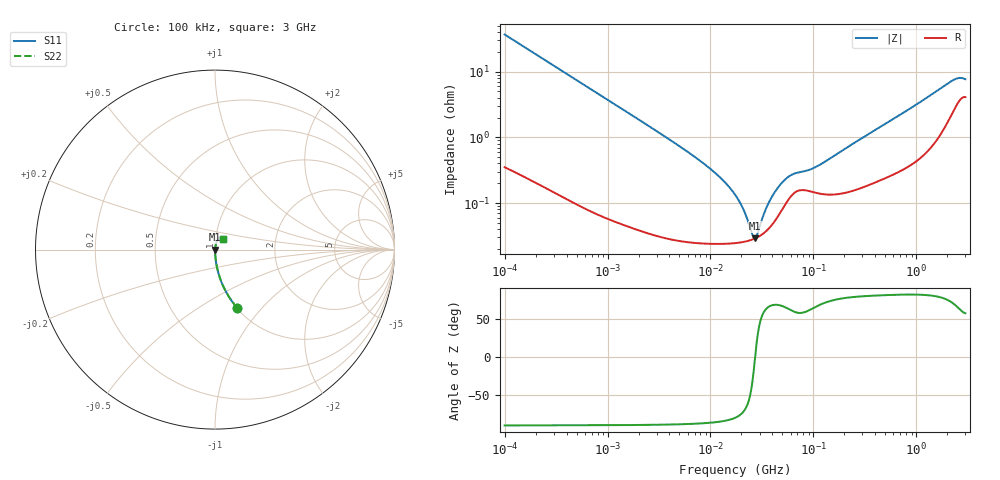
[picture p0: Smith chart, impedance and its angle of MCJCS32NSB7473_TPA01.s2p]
! MCJCS32NSB7473_TPA01  S-PARAMETER MODEL  ( Standard Model )
! Model Generated by TAIYO YUDEN Corporation (http://www.ty-top.com)
! Version 1.0
! TAIYO YUDEN Control No. 220601
! Copyright(c) 2015 TAIYO YUDEN CO.,LTD. All Rights Reserved.
! Product Description (link to TY-COMPAS)
! https://ds.yuden.co.jp/TYCOMPAS/or/detail?pn=MCJCS32NSB7473KTPA01&u=M
! Products Name : Multilayer Ceramic Capacitors
! Characteristics :
!  Capacitance : 0.047 [uF] , Rated Voltage : 630 [V] , TCC : X7R
!  Case Size : 3.2 x 2.5 / 0.126 x 0.098 [mm/inch] , Thickness : 1.9 / 0.075 [mm/inch]
!  (Conditions: Temperature = 25 [degC] , DC Bias Voltage = 0 [V])
! External Node Assignments :
!  1  o---| |---o  2
! GND o---------o GND
! Frequency Range : 100kHz  -  3GHz  [ 401 STEP ]
# MHZ S RI R 50
! Freq[MHz].  S11 Real  S11 Imag  S21 Real  S21 Imag  S12 Real  S12 Imag  S22 Real  S22 Imag
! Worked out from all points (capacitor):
!   401 points, 100 kHz to 3 GHz, reference 50 ohm
!   read as one part in series: C = 43 nF near 105.3 kHz
!   lowest |Z| = 28.8 mohm at 26.84 MHz (marker M1)
!   series resonance near 27.15 MHz, so ESL is about 800 pH
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0.1  0.1224 -0.323  0.8776 0.323  0.8776 0.323  0.1224 -0.323
0.234079  0.0262 -0.1543  0.9738 0.1543  0.9738 0.1543  0.0262 -0.1543
0.562235  0.00525 -0.0661  0.9947 0.0661  0.9947 0.0661  0.00525 -0.0661
3.161081  0.000447 -0.0118  0.9996 0.0118  0.9996 0.0118  0.000447 -0.0118
6.3393  0.000282 -0.00566  0.9997 0.00566  0.9997 0.00566  0.000282 -0.00566
10.08119  0.000249 -0.00326  0.9998 0.00326  0.9998 0.00326  0.000249 -0.00326
14.09348  0.000243 -0.00199  0.9998 0.00199  0.9998 0.00199  0.000243 -0.00199
17.7727  0.000247 -0.00124  0.9998 0.00124  0.9998 0.00124  0.000247 -0.00124
20.74485  0.000255 -0.00078  0.9997 0.00078  0.9997 0.00078  0.000255 -0.00078
25.49486  0.000277 -0.000183  0.9997 0.000183  0.9997 0.000183  0.000277 -0.000183
26.84345  0.000286 -3.32e-05  0.9997 3.32e-05  0.9997 3.32e-05  0.000286 -3.32e-05
28.26337  0.000297 0.000117  0.9997 -0.000117  0.9997 -0.000117  0.000297 0.000117
32.98988  0.000347 0.00058  0.9997 -0.00058  0.9997 -0.00058  0.000347 0.00058
37.52708  0.000421 0.000984  0.9996 -0.000984  0.9996 -0.000984  0.000421 0.000984
42.68829  0.000546 0.0014  0.9995 -0.0014  0.9995 -0.0014  0.000546 0.0014
48.55934  0.000749 0.00182  0.9993 -0.00182  0.9993 -0.00182  0.000749 0.00182
62.83488  0.00135 0.00238  0.9987 -0.00238  0.9987 -0.00238  0.00135 0.00238
97.38194  0.00148 0.00298  0.9985 -0.00298  0.9985 -0.00298  0.00148 0.00298
547.5153  0.00283 0.0172  0.9972 -0.0172  0.9972 -0.0172  0.00283 0.0172
2201.951  0.0261 0.0655  0.9739 -0.0655  0.9739 -0.0655  0.0261 0.0655
2570.185  0.038 0.0671  0.962 -0.0671  0.962 -0.0671  0.038 0.0671
3000  0.0432 0.0597  0.9568 -0.0597  0.9568 -0.0597  0.0432 0.0597
